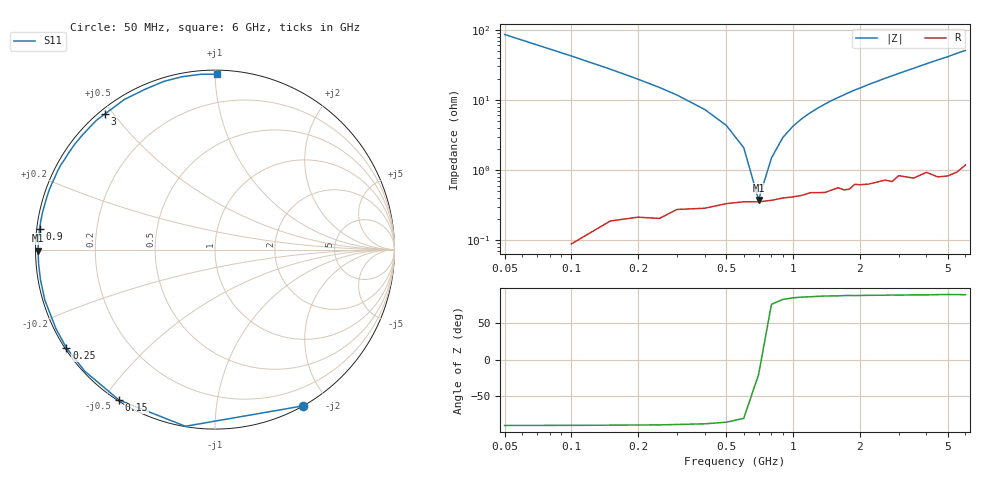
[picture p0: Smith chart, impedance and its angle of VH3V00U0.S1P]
! Infineon Technologies  Discrete & RF Semiconductors
! BB 814
! Si Tuning Diode in SOT23
! VR = 3 V
! S-Parameters:  July  1999
# GHz  S  MA  R  50
!  f  S11
! GHz  MAG  ANG
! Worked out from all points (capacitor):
!   34 points, 50 MHz to 6 GHz, reference 50 ohm
!   read as one part to ground: C = 36.9 pF near 50 MHz
!   lowest |Z| = 376 mohm at 700 MHz (marker M1)
!   series resonance near 708.3 MHz, so ESL is about 1.4 nH
!   S11 on the Smith chart (normalised r, x): 50 MHz: 0.00, -1.71; 150 MHz: 0.00, -0.55; 250 MHz: 0.00, -0.30; 900 MHz: 0.01, +0.06; 3 GHz: 0.02, +0.48; 6 GHz: 0.02, +1.01
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0.05  1 -60.5
0.1  0.9979 -99.5
0.15  0.9942 -122.5
0.2  0.9927 -136.9
0.25  0.9925 -146.5
0.3  0.9897 -153.6
0.4  0.9889 -163.4
0.5  0.9869 -170.1
0.6  0.986 -175.3
0.7  0.986 -179.7
0.8  0.9853 176.7
0.9  0.9842 173.4
1.1  0.9829 167.6
1.2  0.9814 165.0
1.5  0.9801 157.7
1.6  0.9788 155.6
1.9  0.9769 149.1
2.2  0.9775 143.2
2.4  0.9765 139.6
2.6  0.9756 135.8
2.8  0.9773 132.5
3  0.9732 129.0
3.5  0.977 121.1
4  0.9744 113.6
4.5  0.9796 106.8
5  0.9806 100.8
5.5  0.98 94.4
6  0.977 89.2
